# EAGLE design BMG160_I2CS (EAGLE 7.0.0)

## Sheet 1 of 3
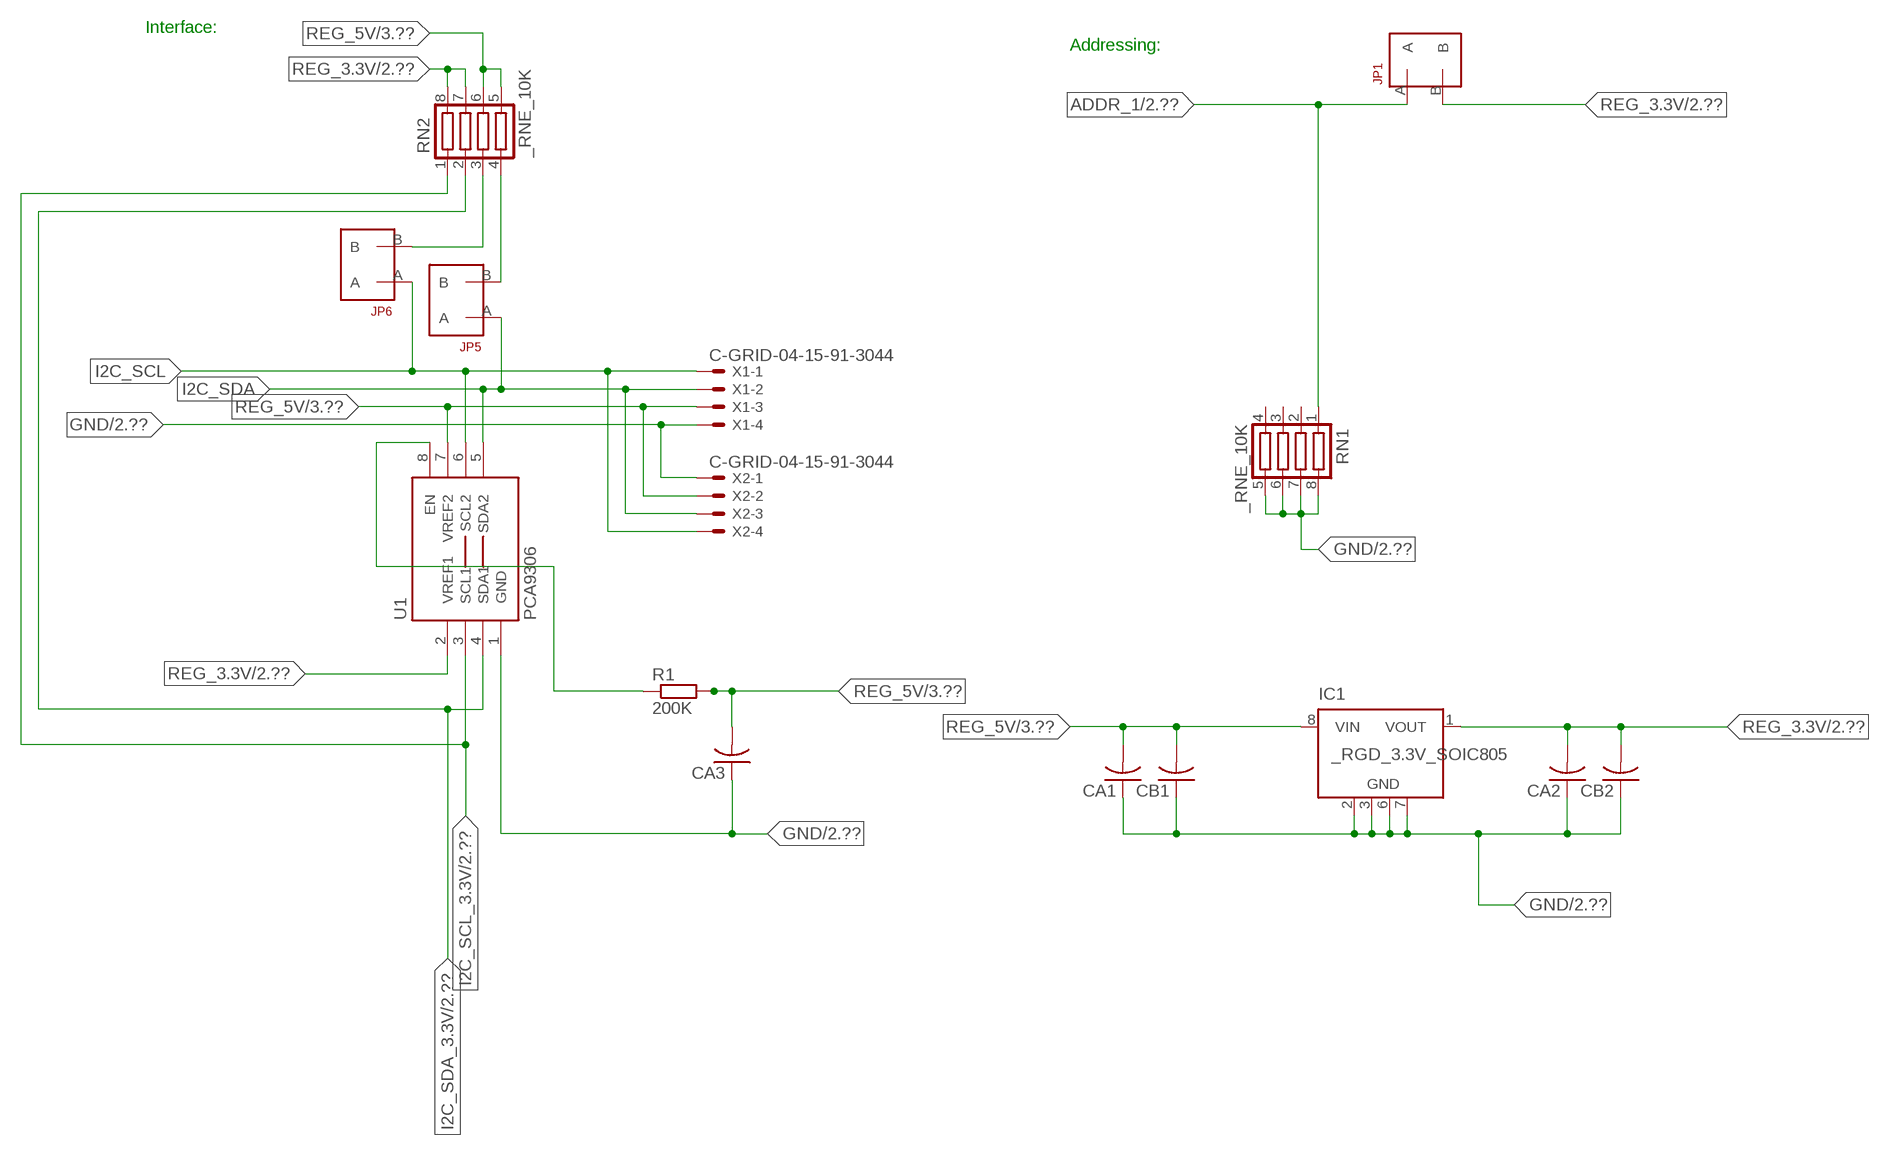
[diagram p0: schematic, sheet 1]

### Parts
CA1  CC1206KRX7R9BB104  [.1UF]
CA2  CC1206KRX7R9BB104  [.1UF]
CA3  CC1206KRX7R9BB104  [.1UF]
CB1  TMK316F106ZL-TC1206K  [TMK316F106ZL-T]
CB2  TMK316F106ZL-TC1206K  [TMK316F106ZL-T]
IC1  _RGD_3.3V_SOIC805  [_RGC_3.3V_SOIC8]
JP1  JUMPER_1X2_2MM  [JUMPER_1X2_2MM]
JP5  JUMPER_1X2_2MM  [JUMPER_1X2_2MM]
JP6  JUMPER_1X2_2MM  [JUMPER_1X2_2MM]
R1  200K  RESISTOR_SMT-0603  [R603]
RN1  _RNE_10K  [RNE]
RN2  _RNE_10K  [RNE]
U1  PCA9306  PCA9306_NCD  [PSOP-8]
X1  C-GRID-04-15-91-3044  [15-91-04]
X2  C-GRID-04-15-91-3044  [15-91-04]

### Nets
ADDR_1: JP1.A RN1.1 ; also sheet 2
GND: CA1.1 CA2.1 CA3.1 CB1.1 CB2.1 IC1.2(GND) IC1.3(GND) IC1.6(GND) IC1.7(GND) RN1.5 RN1.6 RN1.7 RN1.8 U1.1(GND) X1.4 X2.1 ; also sheet 2,3
I2C_SCL: JP6.A U1.6(SCL2) X1.1 X2.4
I2C_SCL_3.3V: RN2.1 U1.3(SCL1) ; also sheet 2
I2C_SDA: JP5.A U1.5(SDA2) X1.2 X2.3
I2C_SDA_3.3V: RN2.2 U1.4(SDA1) ; also sheet 2
N$1: JP6.B RN2.3
N$2: JP5.B RN2.4
N$3: R1.1 U1.8(EN)
REG_3.3V: CA2.2 CB2.2 IC1.1(VOUT) JP1.B RN2.7 RN2.8 U1.2(VREF1) ; also sheet 2
REG_5V: CA1.2 CA3.2 CB1.2 IC1.8(VIN) R1.2 RN2.5 RN2.6 U1.7(VREF2) X1.3 X2.2 ; also sheet 3
Unconnected: IC1.4(NC) IC1.5(NC) RN1.2 RN1.3 RN1.4

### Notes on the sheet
- Interface:
- Addressing:

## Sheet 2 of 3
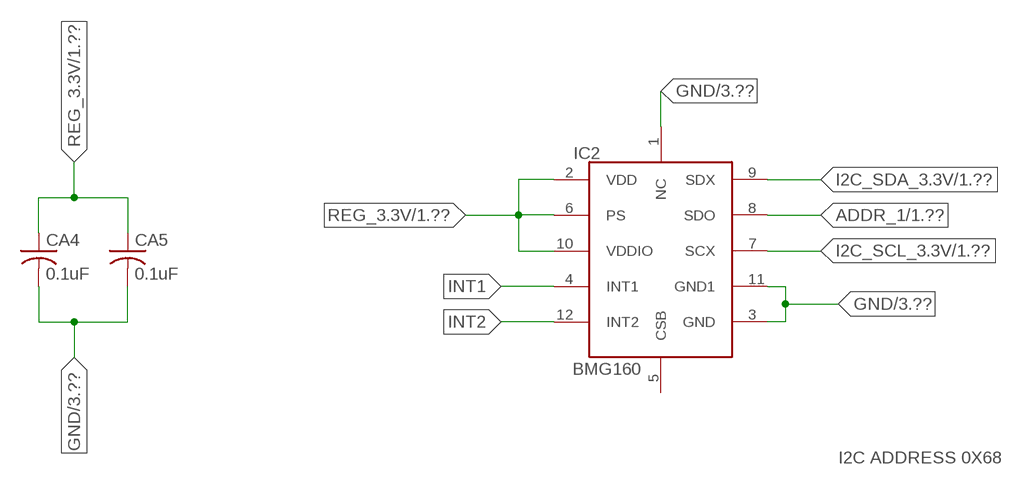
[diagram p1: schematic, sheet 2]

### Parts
CA4  0.1uF  CC1206KRX7R9BB104C1206K  [CC1206KRX7R9BB104]
CA5  0.1uF  CC1206KRX7R9BB104C1206K  [CC1206KRX7R9BB104]
IC2  BMG160  [BMG160]

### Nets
ADDR_1: IC2.8(SDO) ; also sheet 1
GND: CA4.2 CA5.2 IC2.1(NC) IC2.3(GND) IC2.11(GND1) ; also sheet 1,3
I2C_SCL_3.3V: IC2.7(SCX) ; also sheet 1
I2C_SDA_3.3V: IC2.9(SDX) ; also sheet 1
INT1: IC2.4(INT1)
INT2: IC2.12(INT2)
REG_3.3V: CA4.1 CA5.1 IC2.2(VDD) IC2.6(PS) IC2.10(VDDIO) ; also sheet 1
Unconnected: IC2.5(CSB)

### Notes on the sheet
- I2C ADDRESS 0X68

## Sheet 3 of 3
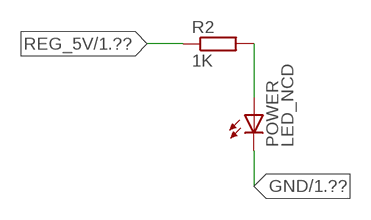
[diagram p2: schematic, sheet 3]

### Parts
POWER  LED_NCD  [CHIPLED_0603]
R2  1K  RESISTOR_SMT-0402  [R402]

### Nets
GND: POWER.C ; also sheet 1,2
N$4: POWER.A R2.2
REG_5V: R2.1 ; also sheet 1

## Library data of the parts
CA1-CA3 = NCD_ULTIMATE_LIBRARY:CC1206KRX7R9BB104: Capacitor CA .1uF 50V SMT C1206K CC1206KRX7R9BB104
CA4 CA5 = NCD_ULTIMATE_LIBRARY (1):CC1206KRX7R9BB104: Capacitor CA .1uF 50V SMT C1206K CC1206KRX7R9BB104
CB1 CB2 = NCD_ULTIMATE_LIBRARY:TMK316F106ZL-T: Capacitor CB 10uF SMT 1206 TMK316F106ZL-T
IC1 = NCD_ULTIMATE_LIBRARY:_RGD_3.3V_SOIC8: Regulator Linear 3.3V Chip Positive VOLTAGE REGULATOR Digikey 497-1199-2-ND/L78L33ACD13TR
IC2 = NCD_ULTIMATE_AMAN:BMG160
JP1 JP5 JP6 = NCD_ULTIMATE_CONNECTORS:JUMPER_1X2_2MM
POWER = NCD_ULTIMATE_LIBRARY:LED_NCD: LED Digikey 754-1132-2-ND/APT2012SRCPRV
R1 R2 = NCD_ULTIMATE_LIBRARY:RESISTOR_SMT: NCD Resistor
RN1 RN2 = NCD_ULTIMATE_LIBRARY:_RNE_10K: Resistor Array RNE SMT 10K x 4 Single Resistor Source: http://www.ctscorp.com/components/Datasheets/CTSChipArrayDs.pdf Digikey 742C083103JPTR-ND/742C083103JP; OC_FARNELL: unknown; OC_NEWARK: unknown
U1 = NCD_ULTIMATE_LIBRARY:PCA9306_NCD: NCD Bidirectional I2C level shifter. NOT compatible with all available part number pinout schemes- DOUBLE CHECK!!!; PROD_ID: IC-10023
X1 X2 = NCD_ULTIMATE_CONNECTORS:C-GRID-04: CONNECTOR 4-Pos I2C wire to board 2.54 mm (0.100") pitch header Digikey WM1342-ND/0015912045; OC_FARNELL: unknown; OC_NEWARK: unknown

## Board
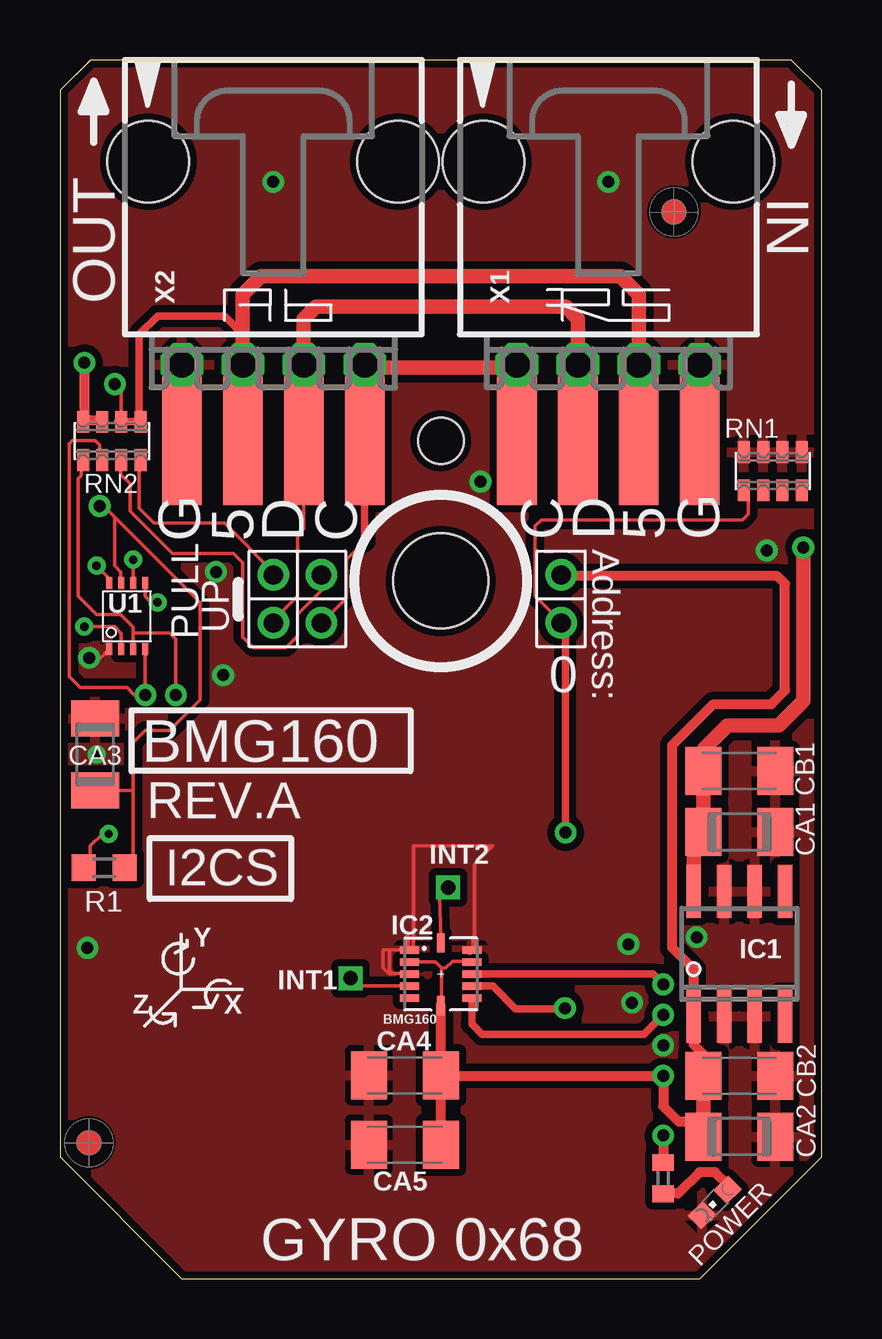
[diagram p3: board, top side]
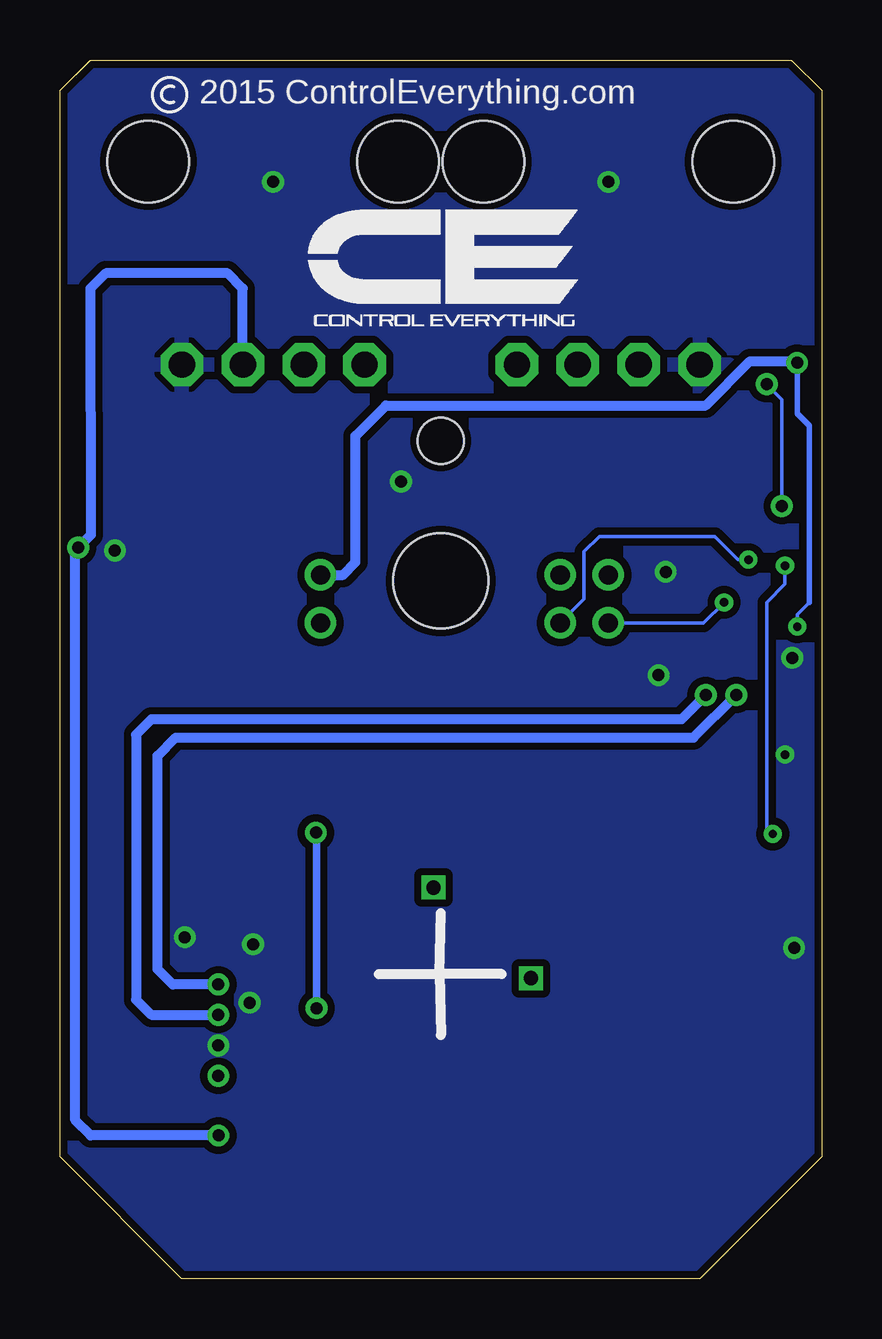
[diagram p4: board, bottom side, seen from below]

Size 31.75 x 50.8 mm. Coordinates in mm from the lower left corner, seen from the top.
Outline: 31.75,5.08 31.75,49.53 30.48,50.8 1.27,50.8 0,49.53 0,5.08 5.08,0 26.67,0 31.75,5.08
Outline: 31.75,5.08 31.75,49.53 30.48,50.8 1.27,50.8 0,49.53 0,5.08 5.08,0 26.67,0 31.75,5.08
Copper layers (1*16): Top 0.035mm / dielectric 1.5mm / Bottom 0.035mm
Design rules "default": minimum track width 5mil, minimum drill 24mil, track to track 5mil, track to pad 5mil, pad to pad 5mil, via to via 5mil, smd to smd 5mil, copper to edge 10mil, drill to drill 8mil, minimum pad ring 10mil, minimum via ring 8mil, stop-mask expansion 2mil, vias tented up to drill 0mil, thermal gap 10mil
Holes 3.96 mm at 15.88,29.08
Holes 1.91 mm at 15.88,34.93

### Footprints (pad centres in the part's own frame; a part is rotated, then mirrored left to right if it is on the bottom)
.1UF = smd 1.5 x 2: 1 -1.5,0; 2 1.5,0
CC1206KRX7R9BB104 = smd 1.5 x 2: 1 -1.5,0; 2 1.5,0
TMK316F106ZL-T = smd 1.5 x 2: 1 -1.5,0; 2 1.5,0
_RGC_3.3V_SOIC8 = smd 0.6 x 2.2: 1 -1.905,-2.6; 2 -0.635,-2.6; 3 0.635,-2.6; 4 1.905,-2.6; 5 1.905,2.6; 6 0.635,2.6; 7 -0.635,2.6; 8 -1.905,2.6
BMG160 = smd 0.8 x 0.32: 1 -1.3,1; 2 -1.3,0.5; 3 -1.3,0; 4 -1.3,-0.5; 5 -1.3,-1; 7 1.3,-1; 8 1.3,-0.5; 9 1.3,0; 10 1.3,0.5; 11 1.3,1 | smd 0.32 x 0.8: 6 0,-1.3; 12 0,1.3
JUMPER_1X2_2MM = drill 0.8: A 0,2; B 0,0
CHIPLED_0603 = smd 0.8 x 0.876: A 0,-0.75; C 0,0.75
R603 = smd 1 x 1.1: 1 -0.85,0; 2 0.85,0
R402 = smd 0.7 x 0.9: 1 -0.65,0; 2 0.65,0
RNE = smd 0.5 x 0.9: 1 -1.2,-0.8; 2 -0.4,-0.8; 3 0.4,-0.8; 4 1.2,-0.8; 5 1.2,0.8; 6 0.4,0.8; 7 -0.4,0.8; 8 -1.2,0.8
PSOP-8 = smd 0.25 x 0.5: 1 -0.73,-1.37; 2 -0.23,-1.37; 3 0.27,-1.37; 4 0.77,-1.37; 5 0.77,1.38; 6 0.27,1.38; 7 -0.23,1.38; 8 -0.73,1.38
15-91-04 = drill 1.1 pad 1.778 octagon: 1 -3.81,-7.62; 2 -1.27,-7.62; 3 1.27,-7.62; 4 3.81,-7.62 | smd 1.651 x 5.334: P1 -3.81,-10.795; P2 -1.27,-10.795; P3 1.27,-10.795; P4 3.81,-10.795 | hole 3.404: -5.207,0.838; 5.207,0.838

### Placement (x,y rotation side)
CA1  28.32,18.62 180 top
CA2  28.32,5.92 180 top
CA3  1.46,21.86 270 top
CA4  14.38,8.48 180 top
CA5  14.38,5.59 180 top
CB1  28.32,21.16 180 top
CB2  28.32,8.46 180 top
IC1  28.32,13.54 0 top
IC2  15.88,12.7 0 top
JP1  20.89,29.34 180 top
JP5  8.89,29.34 180 top
JP6  10.9,29.34 180 top
POWER  27.3,3.18 135 top
R1  1.84,17.13 0 top
R2  25.15,4.19 270 top
RN1  29.72,33.66 0 top
RN2  2.16,34.93 0 top
U1  2.79,27.61 0 top
U$5  [VISION_REF10]  1.21,5.66 90 top
U$28  [VISION_REF10]  25.59,44.46 90 top
X1  22.86,45.72 0 top
X2  8.89,45.72 0 top

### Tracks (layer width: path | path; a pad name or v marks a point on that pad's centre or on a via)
ADDR_1  (via drill 0.5)
  Top 0.152: JP1.A 20.89,27.37 19.81,28.45 19.81,31.37 20.07,31.62 28.45,31.62 28.7,31.88 28.7,32.78 RN1.1
  Top 0.305: IC2.8 18.05,12.2 19,11.25 21.03,11.25 v21.06,11.28 | v21.08,18.59 21.08,27.15 JP1.A
  Bottom 0.305: v21.06,11.28 21.06,18.57 v21.08,18.59
GND  (via drill 0.35, 0.5)
  Top 0.152: CA3.1 1.52,23.42 1.52,23.62 | U1.1 1.7,25.88 v1.22,25.88 | 14.66,13.67 14.63,13.64 IC2.1 13.83,13.7 13.74,13.61 13.74,12.85 13.87,12.73 | IC2.3 14.55,12.73 13.87,12.73 | IC2.11 17.09,13.61 | 13.87,12.73 13.84,12.7 13.72,12.7 13.46,12.95 13.46,13.72 14.73,13.72 14.73,18.03 18.03,18.03 17.27,17.27 17.27,14.22
  Top 0.254: 17.09,13.61 17.27,13.8 17.27,14.22 | 14.66,13.67 14.48,13.85 14.48,14.22
  other vias: 8.89,45.72 22.86,45.72 25.15,9.73 6.8,25.16 17.53,33.22 26.55,14.24 1.15,13.79 6.5,29.46 1.52,21.84 23.85,11.51 23.7,13.94 29.46,30.35
  pour Top (isolate 0.305): -1.27,0 -1.27,50.8 33.02,50.8 33.02,0
  pour Bottom (isolate 0.305): -5.08,0 -5.08,50.8 35.56,50.8 35.56,0
I2C_SCL  (via drill 0.35)
  Top 0.152: 12.7,30.73 11.94,29.97 11.94,28.38 JP6.A | v3.05,29.97 3.06,29.96 U1.6
  Top 0.305: 12.7,30.73 X2.4
  Top 0.406: X2.4 12.7,37.97 | 19.05,37.97 X1.1
  Top 0.61: 12.7,37.97 19.05,37.97
  Bottom 0.152: JP6.A 9.91,28.33 9.91,30.3 9.27,30.94 4.45,30.94 3.48,29.97 v3.05,29.97
I2C_SCL_3.3V  (via drill 0.5)
  Top 0.152: RN2.1 0.89,34.07 0.89,33.48 0.77,33.35 0.77,29.1 0.76,29.09 0.76,28.45 1.52,27.69 2.54,27.69 3.06,27.17 3.06,26.92 | 3.06,26.92 U1.3 | v4.83,24.33 v4.83,24.34 4.83,26.67 4.57,26.92 3.06,26.92
  Top 0.305: IC2.7 17.18,10.61 17.6,10.19 24.34,10.19 v25.15,11
  Bottom 0.406: v4.83,24.33 5.84,23.32 27.94,23.32 28.58,22.68 28.58,11.63 27.94,11 v25.15,11
I2C_SDA  (via drill 0.35)
  Top 0.152: JP5.A 8.89,27.44 9.91,28.45 9.91,30.99 10.16,31.24 10.16,34.92 X2.3 | U1.5 3.56,28.45 3.81,28.19 v4.06,28.19
  Top 0.305: 10.35,34.73 X2.3
  Top 0.61: X2.3 10.16,40.01 10.67,40.51 21.09,40.51 21.59,40.01 X1.2
  Bottom 0.152: v4.06,28.19 4.92,27.34 JP5.A
I2C_SDA_3.3V  (via drill 0.5)
  Top 0.152: RN2.2 1.65,34.14 1.65,34.75 1.46,34.94 0.51,34.94 0.38,34.81 0.38,26.37 0.38,26.36 0.38,25.1 0.84,24.64 2.79,24.64 3.1,24.33 v3.56,24.33 v3.56,24.34 U1.4
  Top 0.305: IC2.9 24.72,12.7 v25.15,12.27
  Bottom 0.406: v25.15,12.27 27.05,12.27 27.69,12.9 27.69,21.79 26.93,22.56 5.34,22.56 v3.56,24.33
INT1  (via drill 0.6)
  Top 0.152: v12.12,12.52 12.44,12.2 IC2.4
INT2  (via drill 0.6)
  Top 0.152: v16.18,16.31 15.82,15.95 15.88,14.17 IC2.12
N$1
  Top 0.152: JP6.B 10.92,29.31 10.92,28.7 9.91,27.69 9.91,26.8 9.42,26.31 8.06,26.31 7.62,26.75 7.62,29.84 7.24,30.23 4.7,30.23 2.92,32 2.92,33.15 2.54,33.53 2.54,34.1 RN2.3
  Top 0.305: 2.54,34.02 RN2.3
N$2
  Top 0.152: JP5.B 8.89,29.46 6.86,31.5 3.94,31.5 3.3,32.13 3.3,34.07 RN2.4
  Top 0.305: 3.37,33.88 RN2.4
N$3  (via drill 0.35)
  Top 0.152: R1.1 1.27,17.41 1.27,18.03 1.78,18.54 v2.03,18.54 | v1.52,29.72 2.06,29.18 U1.8
  Bottom 0.152: v2.03,18.54 2.29,18.8 2.29,28.19 1.52,28.96 v1.52,29.72
N$4
  Top 0.406: POWER.A 27.84,3.92 27.3,4.45 26.67,4.45 25.78,3.56 25.16,3.56 R2.2
REG_3.3V  (via drill 0.35, 0.5)
  Top 0.152: v1.02,27.18 2.29,27.18 2.56,26.9 U1.2 | IC2.6 15.9,11.43 15.9,12.95 | 15.9,12.95 15.65,13.2 IC2.2 | IC2.10 17.14,13.23 16.36,13.23 16.08,12.95 15.9,12.95
  Top 0.406: CB2.2 26.82,9.35 26.42,9.75 26.42,10.36 | 26.82,6.55 25.78,6.55 25.15,7.19 v25.15,8.46 15.9,8.46 CA4.1 | IC1.1 26.42,12.9 25.53,13.79 25.53,22.24 27.24,23.95 29.66,23.95 30.23,24.52 30.23,28.97 29.91,29.29 20.89,29.29 JP1.B | 26.52,5.62 CA2.2 | v1.02,38.18 1.02,35.78 | 1.02,35.78 RN2.8 | 1.02,35.78 1.71,35.78 RN2.7 | CA5.1 CA4.1 | CA4.1 IC2.6
  Top 0.61: CB2.2 26.82,6.55 CA2.2 | 26.42,10.36 IC1.1
  Bottom 0.152: 0.51,28.19 1.02,27.69 v1.02,27.18
  Bottom 0.229: 0.51,28.19 0.51,35.56 1.02,36.07 v1.02,38.18
  Bottom 0.406: v1.02,38.18 1.08,38.24 2.99,38.24 4.83,36.4 18.16,36.4 19.43,35.13 19.43,29.87 19.94,29.34 JP1.B
REG_5V  (via drill 0.5)
  Top 0.152: RN2.6 2.56,37.01 v2.29,37.29 | R1.2 3.05,17.49 3.05,20.36 | 3.05,20.36 3.05,22.35 3.56,22.86 4.57,22.86 5.84,24.13 5.84,28.19 2.29,31.75 | CA3.2 3.05,20.36 | 2.29,31.75 1.83,32.21 v1.65,32.21 | U1.7 2.54,29.01 2.54,29.46 2.29,29.72 2.29,31.75
  Top 0.305: 7.62,39.37 7.5,39.37 | 2.42,35.74 RN2.6 RN2.5 3.31,35.8 3.31,39.37 4.07,40.13 6.86,40.13 7.62,39.37 | X2.2 7.62,39.37
  Top 0.406: v25.15,5.97 R2.1
  Top 0.61: X2.2 7.62,41.02 8.38,41.78 23.37,41.78 24.13,41.02 X1.3 | IC1.8 26.42,18.21 CA1.2 CB1.2 26.86,21.2 26.86,22.11 27.82,23.06 29.98,23.06 30.99,24.08 v30.99,30.48
  Bottom 0.152: v1.65,32.21 1.65,36.65 v2.29,37.29
  Bottom 0.406: X1.3 24.13,41.28 24.77,41.91 29.84,41.91 30.48,41.27 30.47,31 v30.99,30.48 31.11,30.36 31.11,6.6 30.48,5.97 v25.15,5.97

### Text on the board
tPlace: Y | Z | X
tNames: IN | OUT | G | 5 | D | C | C | D | 5 | G | Address: | PULL | UP | 0 | BMG160 | REV.A | INT2 | I2CS | INT1 | GYRO 0x68
bNames: 2015 ControlEverything.com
